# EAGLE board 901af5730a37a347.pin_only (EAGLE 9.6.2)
REV: B

Size 25.4 x 17.78 mm. Coordinates in mm from the lower left corner, seen from the top.
Outline: 0,15.24 0,2.54 arc90 2.54,0 22.86,0 arc90 25.4,2.54 25.4,15.24 arc90 22.86,17.78 2.54,17.78 arc90 0,15.24
Copper layers (1*16): Top 0.035mm / dielectric 1.5mm / Bottom 0.035mm
Design rules "adafruit *": minimum track width 8mil, minimum drill 15.5mil, track to track 8mil, track to pad 8mil, pad to pad 8mil, via to via 8mil, smd to smd 8mil, copper to edge 10mil, drill to drill 8mil, minimum pad ring 10mil, minimum via ring 8mil, stop-mask expansion 2mil, vias tented up to drill 20mil, thermal gap 10mil
Net classes: 1 highpower: width 0.305 mm, drill 0.483 mm; 2 lowpower: width 0.254 mm, drill 0.483 mm

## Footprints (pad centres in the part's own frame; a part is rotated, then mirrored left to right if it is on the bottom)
0603-NO = smd 1.075 x 1: 1 -0.85,0; 2 0.85,0
0805-NO = smd 1.24 x 1.5: 1 -0.95,0; 2 0.95,0
JST_SH4 = smd 0.6 x 1.55: 1 -1.5,2.514; 2 -0.5,2.514; 3 0.5,2.514; 4 1.5,2.514 | smd 1.2 x 1.8: MT1 -2.8,-1.386; MT2 2.8,-1.386
CHIPLED_0603_NOOUTLINE = smd 0.8 x 0.8: A 0,-0.75; C 0,0.75
FIDUCIAL_1MM = smd 1 x 1: 1 0,0
1X06_ROUND_70 = drill 1 pad 1.778: 1 -6.35,0; 2 -3.81,0; 3 -1.27,0; 4 1.27,0; 5 3.81,0; 6 6.35,0
SOT363 = smd 0.5 x 0.5: 1 -0.75,-0.9; 3 0.75,-0.9; 4 0.75,0.9; 6 -0.75,0.9 | smd 0.4 x 0.5: 2 0,-0.9; 5 0,0.9
RESPACK_4X0603 = smd 0.45 x 0.9: 1 -1.3,-0.85; 2 -0.4,-0.85; 3 0.4,-0.85; 4 1.3,-0.85; 5 1.3,0.85; 6 0.4,0.85; 7 -0.4,0.85; 8 -1.3,0.85
DFN6_TAOS = smd 1.2 x 0.35: 1 -0.8,0.65; 2 -0.8,0; 3 -0.8,-0.65; 4 0.8,-0.65; 5 0.8,0; 6 0.8,0.65
SOT23-5 = smd 0.55 x 1.2: 1 -0.95,-1.3; 2 0,-1.3; 3 0.95,-1.3; 4 0.95,1.3; 5 -0.95,1.3
MOUNTINGHOLE_2.5_PLATED = drill 2.5 pad 3.2: P$1 0,0

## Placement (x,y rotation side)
C1  0.1uF  [0603-NO]  11.81,5.71 0 top
C2  10uF  [0805-NO]  7.87,5.71 0 top
C3  10uF  [0805-NO]  8.13,12.19 0 top
CONN3  STEMMA_I2C_QT  [JST_SH4]  22.73,8.89 90 top
CONN4  STEMMA_I2C_QT  [JST_SH4]  2.67,8.89 270 top
D1  GREEN  [CHIPLED_0603_NOOUTLINE]  3.56,12.57 90 top
FID3  FIDUCIAL_1MM  [FIDUCIAL_1MM]  5.21,4.83 0 top
FID4  FIDUCIAL_1MM  [FIDUCIAL_1MM]  19.56,16.51 0 top
JP1  [1X06_ROUND_70]  12.7,2.54 0 top
Q2  BSS138  [SOT363]  16.89,7.49 90 top
R1  10K  [0603-NO]  5.59,12.45 270 top
R3  10K  [RESPACK_4X0603]  17.14,11.43 180 top
U1  TSL2591  [DFN6_TAOS]  12.7,8.89 180 top
U2  AP2112K-3.3  [SOT23-5]  8.13,8.76 0 top
U$1  MOUNTINGHOLE2.5  [MOUNTINGHOLE_2.5_PLATED]  2.54,15.24 0 top
U$17  MOUNTINGHOLE2.5  [MOUNTINGHOLE_2.5_PLATED]  22.86,15.24 0 top
U$19  MOUNTINGHOLE2.5  [MOUNTINGHOLE_2.5_PLATED]  2.54,2.54 0 top
U$21  MOUNTINGHOLE2.5  [MOUNTINGHOLE_2.5_PLATED]  22.86,2.54 0 top
U$22  [ADAFRUIT_3.5MM]  4.57,13.72 0 top
U$25  [PCBFEAT-REV-040]  6.1,16.51 0 bottom
U$30  [STEMMAQT]  22.48,4.45 90 bottom
U$31  [STEMMAQT]  2.92,13.34 270 bottom

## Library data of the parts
C1-C3 CONN3 CONN4 D1 JP1 Q2 R1 R3 U1 U2 U$22 U$25 = microbuilder
FID3 FID4 U$1 U$17 U$19 U$21 = microbuilder; BOM: EXCLUDE
U$30 U$31 = silks

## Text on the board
tPlace: TSL2591 | Light Sensor | on | 3Vo | SCL | INT | VIN | GND | SDA
bPlace: TSL2591 | Lux/Light Sensor / IR & Visible / 600M:1 Dynamic Range / Default I2C addr 0x29 | VLogic/Vcc: 3-5VDC

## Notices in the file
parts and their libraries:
microbuilder: This work is placed in the public domain, and may be freely used for commercial and non-commercial work with the following conditions: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
